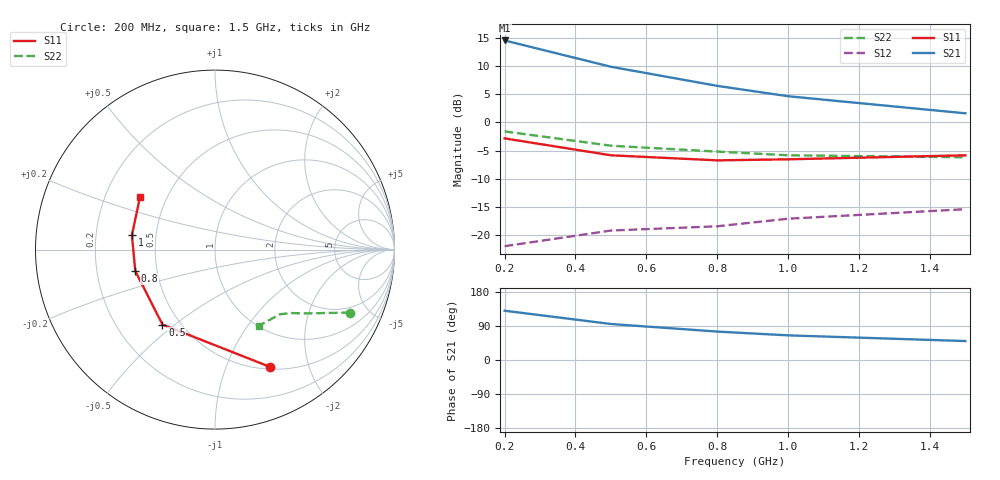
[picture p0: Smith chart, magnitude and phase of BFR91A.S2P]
!  BFR91
!  VCE=5V; IC=2mA
#  GHZ S MA R 50
!  S-PARAMETER DATA
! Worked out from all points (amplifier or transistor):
!   5 points, 200 MHz to 1.5 GHz, reference 50 ohm
!   highest |S21| = 14.5 dB at 200 MHz (marker M1)
!   |S21| within 3 dB of that: start of sweep to 393.2 MHz
!   unconditionally stable (mu >= 1): 804.3 MHz to end of sweep
!   at 200 MHz: K = 0.34, MSG = 18.2 dB, |S12| = -21.9 dB
!   at 800 MHz: K = 1.00, MSG = 12.4 dB, |S12| = -18.4 dB
!   at 1.5 GHz: K = 1.26, MAG = 5.4 dB, |S12| = -15.4 dB
!   S11 on the Smith chart (normalised r, x): 200 MHz: 0.53, -1.43; 500 MHz: 0.40, -0.45; 800 MHz: 0.38, -0.11; 1 GHz: 0.36, +0.08; 1.5 GHz: 0.35, +0.28
0.2  0.72 -65.0  5.3 130.0  0.08 55.0  0.83 -25.0
0.5  0.51 -125.0  3.1 95.0  0.11 45.0  0.62 -35.0
0.8  0.46 -165.0  2.1 75.0  0.12 50.0  0.55 -40.0
1  0.47 170.0  1.7 65.0  0.14 55.0  0.51 -45.0
1.5  0.51 145.0  1.2 50.0  0.17 65.0  0.49 -60.0
